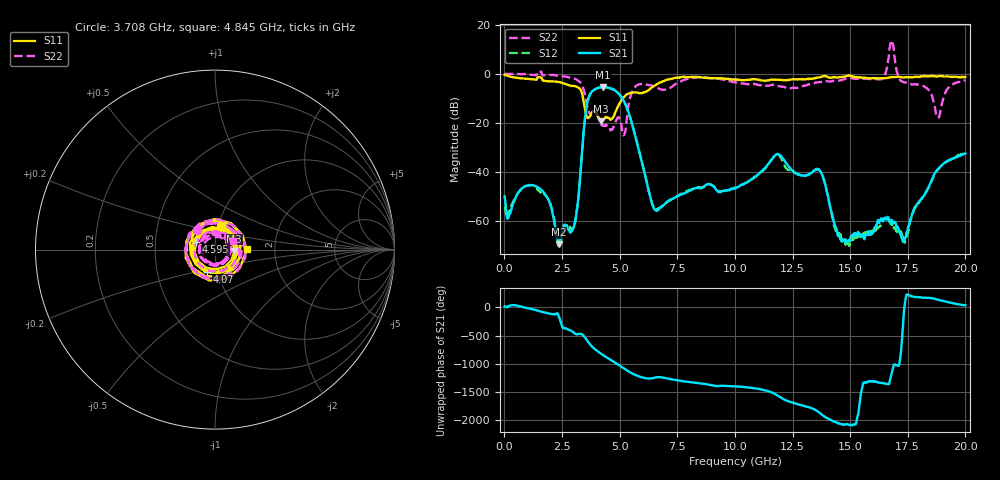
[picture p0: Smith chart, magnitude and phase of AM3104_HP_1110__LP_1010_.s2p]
!Created with skrf (http://scikit-rf.org).
# Hz S RI R 50.0
!freq ReS11 ImS11 ReS21 ImS21 ReS12 ImS12 ReS22 ImS22
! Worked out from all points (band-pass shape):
!   1601 points, 10 MHz to 20 GHz, reference 50 ohm
!   highest |S21| = -5.47 dB at 4.283 GHz (marker M1); lowest = -69.4 dB at 2.359 GHz (marker M2)
!   |S21| within 3 dB of the highest: 3.709 GHz to 4.995 GHz (1.286 GHz wide, 29.6 % of centre)
!   lowest |S11| = -19.3 dB at 4.183 GHz (marker M3), VSWR 1.24, Z = 62 - j1.05 ohm
!   |S11| at or under -10 dB: 3.413 GHz to 5.142 GHz (1.729 GHz wide, 40.4 % of centre)
!   |S22| runs from -25.1 to 13.5 dB; largest |S21 - S12| = 0.045
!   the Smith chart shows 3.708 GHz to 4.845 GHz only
!   S11 on the Smith chart (normalised r, x): 3.708 GHz: 1.03, +0.27; 4.07 GHz: 0.89, -0.22; 4.595 GHz: 0.80, +0.07; 4.845 GHz: 1.43, +0.01
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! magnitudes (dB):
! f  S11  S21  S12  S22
! 10 MHz  -0.4  -49.9  -54.1  0.0
! 1.309 GHz  -2.4  -45.6  -45.6  -0.6
! 2.359 GHz  -3.4  -69.4  -70.2  -0.8
! 3.021 GHz  -5.0  -62.2  -62.0  -1.9
! 3.346 GHz  -7.4  -34.9  -34.9  -4.2
! 3.708 GHz  -17.5  -8.5  -8.6  -16.5
! 4.07 GHz  -17.6  -5.8  -5.8  -18.0
! 4.183 GHz  -19.3  -5.5  -5.6  -20.6
! 4.283 GHz  -18.8  -5.5  -5.5  -21.0
! 4.595 GHz  -18.8  -5.9  -6.0  -22.9
! 4.845 GHz  -15.1  -7.1  -7.2  -19.1
! 5.745 GHz  -7.7  -27.6  -27.7  -4.8
! 6.682 GHz  -4.0  -55.3  -54.8  -6.0
! 10.01 GHz  -2.5  -46.7  -46.7  -3.6
! 11.83 GHz  -2.5  -32.8  -32.9  -4.9
! 13.34 GHz  -2.1  -40.3  -40.2  -4.1
! 14.88 GHz  -0.9  -68.2  -69.2  -1.9
! 16.38 GHz  -1.8  -59.0  -60.8  -2.2
! 16.68 GHz  -1.6  -59.0  -60.0  7.1
! 17.41 GHz  -1.5  -66.5  -68.1  -3.6
! 18.8 GHz  -1.0  -39.0  -39.1  -17.8
! 20 GHz  -1.3  -32.5  -32.1  -2.7
